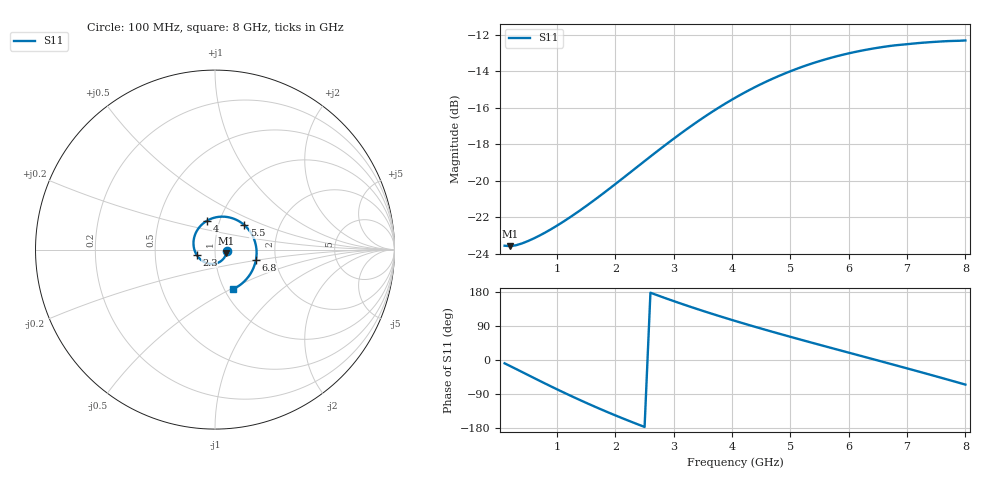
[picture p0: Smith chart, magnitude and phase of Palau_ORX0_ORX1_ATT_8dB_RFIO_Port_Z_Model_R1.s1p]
! Created Fri Oct  9 14:29:27 2020
! Palau ORX0/ORX1 RFIO Port Impedance Model.
! Attenuation  : 8 dB.
! Revision		: R1.
! Impedance Mode 	: Balanced Differential-Mode.
! Impedance Format 	: Series Equivalent Differential Impedance (SEDZ).
# hz S ma R 100
! 1 Port Network Data from SP1.SP block
! freq  magS11  angS11
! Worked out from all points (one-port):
!   80 points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, 100 MHz to 8 GHz, reference 100 ohm
!   lowest |S11| = -23.6 dB at 200 MHz (marker M1), VSWR 1.14, Z = 113 - j4.24 ohm
!   |S11| at or under -10 dB: start of sweep to end of sweep
!   S11 on the Smith chart (normalised r, x): 100 MHz: 1.14, -0.02; 2.3 GHz: 0.81, -0.05; 4 GHz: 0.87, +0.29; 5.5 GHz: 1.33, +0.38; 6.8 GHz: 1.58, -0.19; 8 GHz: 1.10, -0.51
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1e8  0.06629 -8.8
2e8  0.0661 -16.3
4e8  0.06728 -31.7
6e8  0.06941 -47.2
1.1e9  0.07705 -84.8
1.4e9  0.08301 -106.2
1.6e9  0.08753 -120.0
1.8e9  0.09249 -133.3
2.1e9  0.1007 -152.5
2.3e9  0.1068 -164.8
2.7e9  0.1198 171.9
3.1e9  0.134 150.1
3.5e9  0.1486 129.6
4e9  0.1669 105.6
4.1e9  0.1704 100.9
4.4e9  0.1808 87.3
4.6e9  0.1874 78.5
4.8e9  0.1937 69.8
5.1e9  0.2024 56.9
5.5e9  0.2128 40.1
5.8e9  0.2195 27.7
6.1e9  0.2253 15.3
6.5e9  0.2315 -1.3
6.8e9  0.2351 -13.8
7.1e9  0.2377 -26.3
7.5e9  0.2404 -43.3
7.7e9  0.2415 -51.9
8e9  0.2424 -64.9
